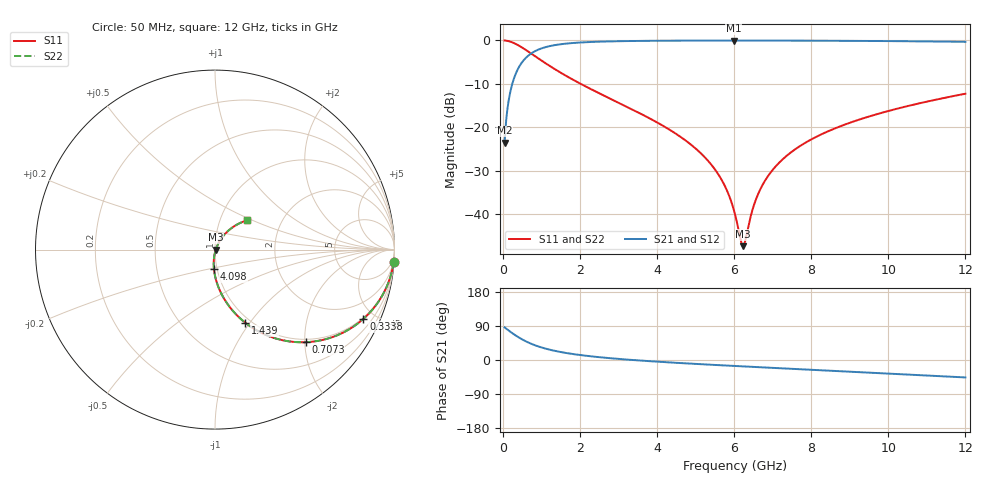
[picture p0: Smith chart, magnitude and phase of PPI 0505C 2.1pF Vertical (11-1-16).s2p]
# GHz S MA R 50
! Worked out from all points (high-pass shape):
!   1601 points, 50 MHz to 12 GHz, reference 50 ohm
!   highest |S21| = -0.04 dB at 5.995 GHz (marker M1); lowest = -23.5 dB at 50 MHz (marker M2)
!   |S21| within 3 dB of the highest: 733.9 MHz to end of sweep
!   lowest |S11| = -47.3 dB at 6.234 GHz (marker M3), VSWR 1.01, Z = 50.4 - j0.127 ohm
!   |S11| at or under -10 dB: 2.024 GHz to end of sweep
!   |S22| runs from -47.3 to 0.0 dB; largest |S21 - S12| = 0
!   S11 on the Smith chart (normalised r, x): 50 MHz: 1, -29; 333.8 MHz: 0.94, -4.31; 707.2 MHz: 0.94, -2.02; 1.439 GHz: 0.94, -0.95; 4.098 GHz: 0.97, -0.21; 12 GHz: 1.35, +0.47
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0.05  0.9978 -4.0  0.06682 86.0  0.06682 86.0  0.9978 -4.0
0.1769688  0.9729 -13.8  0.2308 76.2  0.2308 76.2  0.9729 -13.8
0.3338125  0.9123 -25.0  0.4089 64.9  0.4089 64.9  0.9123 -25.0
0.70725  0.7214 -45.7  0.6912 44.2  0.6912 44.2  0.7214 -45.7
1.043344  0.5715 -57.8  0.8188 32.0  0.8188 32.0  0.5715 -57.8
1.439188  0.4423 -67.4  0.8947 22.3  0.8947 22.3  0.4423 -67.4
2.044156  0.3129 -76.9  0.9472 12.7  0.9472 12.7  0.3129 -76.9
4.038312  0.1118 -92.8  0.99 -4.6  0.99 -4.6  0.1118 -92.8
4.098063  0.108 -93.1  0.9904 -5.0  0.9904 -5.0  0.108 -93.1
5.360281  0.03966 -96.6  0.9949 -12.3  0.9949 -12.3  0.03966 -96.6
5.733719  0.02247 -93.7  0.9953 -14.3  0.9953 -14.3  0.02247 -93.7
5.995125  0.01123 -83.6  0.9953 -15.7  0.9953 -15.7  0.01123 -83.6
6.025  0.01003 -80.9  0.9953 -15.8  0.9953 -15.8  0.01003 -80.9
6.174375  0.005006 -47.7  0.9953 -16.6  0.9953 -16.6  0.005006 -47.7
6.234125  0.00431 -17.0  0.9953 -16.9  0.9953 -16.9  0.00431 -17.0
6.293875  0.005032 13.3  0.9953 -17.2  0.9953 -17.2  0.005032 13.3
6.547813  0.01404 53.1  0.9951 -18.5  0.9951 -18.5  0.01404 53.1
6.846563  0.02615 60.0  0.9947 -20.0  0.9947 -20.0  0.02615 60.0
7.332031  0.04581 61.6  0.9937 -22.4  0.9937 -22.4  0.04581 61.6
8.019156  0.07336 60.2  0.9917 -25.8  0.9917 -25.8  0.07336 60.2
10.01331  0.1548 52.1  0.9813 -35.7  0.9813 -35.7  0.1548 52.1
12  0.2436 42.3  0.962 -46.0  0.962 -46.0  0.2436 42.3
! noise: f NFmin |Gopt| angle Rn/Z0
0.05  0.0008131  0.9467  1.77  0.003416
1.372  0.005596  0.7575  4.915  0.004662
2.701  0.008936  0.7086  8.162  0.006003
4.031  0.01191  0.6798  11.46  0.007127
5.36  0.01475  0.6608  14.75  0.008183
6.682  0.01754  0.6482  17.97  0.00924
8.012  0.02038  0.6404  21.16  0.01036
9.341  0.02334  0.6366  24.3  0.01159
10.67  0.02647  0.6363  27.38  0.01298
12  0.02984  0.6391  30.42  0.01458
